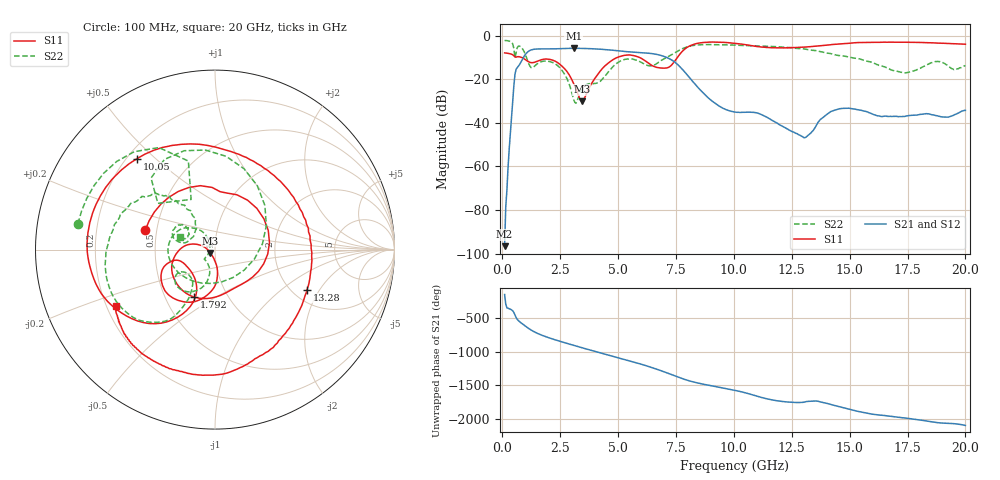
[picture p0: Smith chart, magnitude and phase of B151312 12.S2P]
!  2-Port S-parameters saved by WinCal
! VAR MeasName=S-Parameters (CALIBRATED_DATA) read from VNA (N5244A)
! VAR MeasDate=12/8/2015 5:44:31 PM
! VAR NAME=B151312 12
! VAR FILENAME=B151312 12.S2P
! VAR DATE=12/8/2015 5:44:31 PM
! VAR PHYS_PORTS=1,2
# Hz S DB R 50
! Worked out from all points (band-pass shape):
!   401 points, 100 MHz to 20 GHz, reference 50 ohm
!   highest |S21| = -5.79 dB at 3.085 GHz (marker M1); lowest = -96.6 dB at 100 MHz (marker M2)
!   |S21| within 3 dB of the highest: 986.4 MHz to 6.755 GHz (5.769 GHz wide, 149 % of centre)
!   lowest |S11| = -30.0 dB at 3.433 GHz (marker M3), VSWR 1.07, Z = 47.5 - j1.77 ohm
!   |S11| at or under -10 dB: 839.1 MHz to 4.964 GHz (4.125 GHz wide, 142 % of centre); 5.927 GHz to 7.56 GHz (1.633 GHz wide, 24.2 % of centre)
!   |S22| runs from -31.0 to -2.2 dB; largest |S21 - S12| = 0.0015
!   S11 on the Smith chart (normalised r, x): 100 MHz: 0.43, +0.11; 1.792 GHz: 0.70, -0.40; 10.05 GHz: 0.24, +0.44; 13.28 GHz: 2.39, -1.55; 20 GHz: 0.24, -0.25
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1e8  -7.90 164.2  -96.56 -159.7  -87.63 131.7  -2.19 169.3
5.975e8  -9.84 78.1  -15.37 -139.3  -15.38 -139.3  -7.76 141.0
8.4625e8  -10.03 19.7  -11.28 133.2  -11.28 133.2  -5.62 83.2
1.095e9  -11.71 -35.9  -7.48 70.2  -7.48 70.3  -11.49 7.1
1.3935e9  -12.19 -73.0  -6.20 8.5  -6.20 8.5  -13.97 -110.8
1.7915e9  -10.78 -113.7  -6.06 -50.6  -6.06 -50.6  -11.67 -171.3
2.53775e9  -13.61 -176.4  -5.94 -134.2  -5.94 -134.2  -15.40 135.1
3.085e9  -21.97 163.2  -5.79 170.6  -5.79 170.6  -29.44 147.8
3.43325e9  -30.04 -143.7  -5.84 136.4  -5.84 136.4  -24.67 -142.3
4.08e9  -18.38 -83.4  -6.12 74.3  -6.11 74.3  -21.71 -127.1
4.82625e9  -10.71 -106.7  -6.73 3.9  -6.72 3.9  -13.72 -106.2
5.82125e9  -9.56 -154.7  -7.68 -89.7  -7.66 -89.8  -11.34 -145.2
6.7665e9  -14.72 -150.2  -8.82 167.9  -8.83 167.8  -12.07 -120.7
8.10975e9  -4.63 -137.4  -19.55 4.0  -19.53 4.0  -4.73 -137.6
9.00525e9  -2.93 177.0  -29.53 -63.7  -29.55 -64.2  -4.08 -161.5
1.005e10  -3.51 130.6  -35.03 -133.4  -35.08 -133.5  -4.33 -178.9
1.1443e10  -5.40 66.4  -37.52 101.1  -37.59 101.4  -4.91 164.1
1.328375e10  -5.05 -23.5  -45.04 65.8  -44.98 66.8  -6.58 140.1
1.338325e10  -4.97 -27.3  -43.94 69.0  -43.87 69.3  -6.70 138.2
1.457725e10  -3.84 -67.1  -33.49 -16.9  -33.40 -17.1  -9.12 128.6
1.67165e10  -3.00 -113.5  -37.02 -153.3  -36.85 -153.4  -15.28 128.5
2e10  -3.93 -150.4  -34.26 69.2  -34.27 68.2  -13.70 159.3
